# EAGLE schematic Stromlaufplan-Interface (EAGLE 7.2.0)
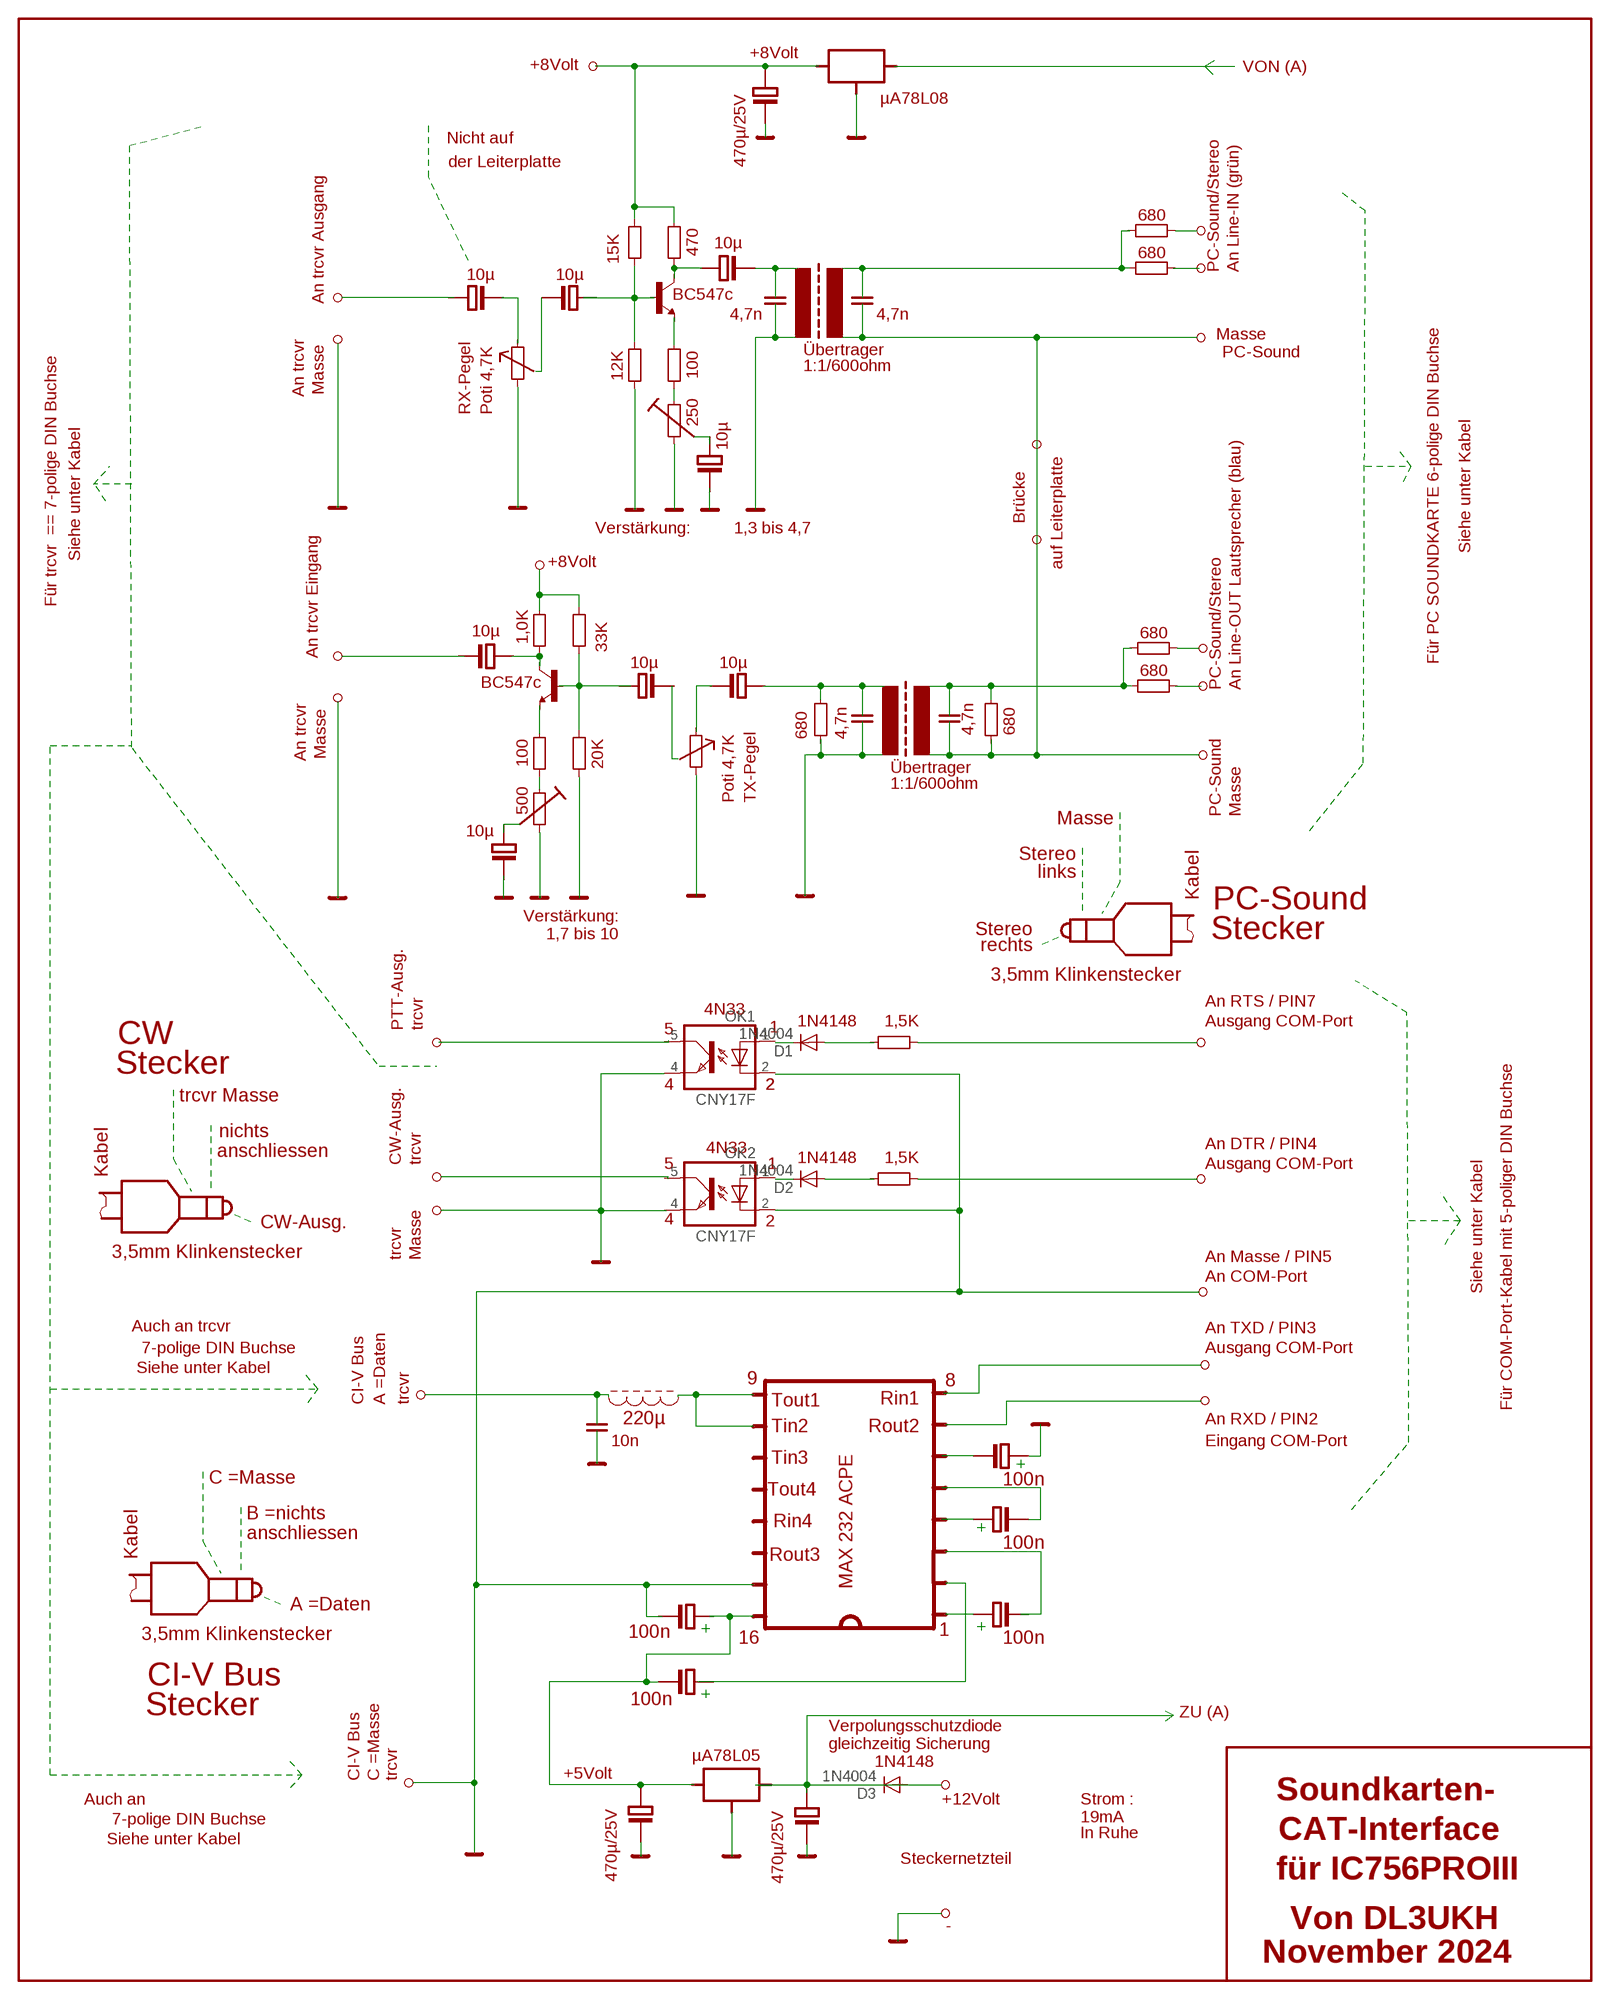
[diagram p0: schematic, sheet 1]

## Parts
D1  1N4004  [DO41-10]
D2  1N4004  [DO41-10]
D3  1N4004  [DO41-10]
OK1  CNY17F  [DIL06]
OK2  CNY17F  [DIL06]

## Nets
N$35: D3.C
N$45: D1.C
N$46: D1.A
N$47: D3.A
N$51: D2.C
N$55: D2.A
Unconnected: OK1.1(A) OK1.2(C) OK1.4(EMIT) OK1.5(COL) OK2.1(A) OK2.2(C) OK2.4(EMIT) OK2.5(COL)

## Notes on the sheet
- +8Volt
- +8Volt | VON (A)
- µA78L08
- Nicht auf
- der Leiterplatte | 470µ/25V
- 680
- 10µ
- 470 | 680
- 15K
- PC-Sound/Stereo | An Line-IN (grün)
- 10µ | 10µ
- An trcvr Ausgang | BC547c
- 4,7n | 4,7n
- Masse
- PC-Sound
- Übertrager
- 1:1/600ohm
- 12K | 100
- An trcvr | Masse
- RX-Pegel | Poti 4,7K
- 250
- 10µ
- Brücke
- Verstärkung: | 1,3 bis 4,7
- Siehe unter Kabel
- Siehe unter Kabel
- +8Volt | auf Leiterplatte
- Für trcvr  == 7-polige DIN Buchse
- 10µ | 680
- 1,0K
- 33K
- An trcvr Eingang
- 10µ | 10µ | Für PC SOUNDKARTE 6-polige DIN Buchse
- 680
- BC547c | PC-Sound/Stereo | An Line-OUT Lautsprecher (blau)
- 680 | 4,7n | 4,7n | 680
- An trcvr | Masse
- 100 | 20K
- Übertrager
- 1:1/600ohm
- Poti 4,7K | TX-Pegel
- 500 | PC-Sound | Masse
- Masse
- 10µ
- Stereo
- links
- Kabel
- PC-Sound
- Verstärkung:
- 1,7 bis 10 | Stereo | Stecker
- rechts
- 3,5mm Klinkenstecker
- An RTS / PIN7
- 4N33
- PTT-Ausg. | trcvr | 1N4148 | 1,5K | Ausgang COM-Port
- 5 | 1
- CW
- Stecker
- 4 | 2 | 2
- trcvr Masse
- nichts
- 4N33 | An DTR / PIN4
- anschliessen
- CW-Ausg. | trcvr | 1N4148 | 1,5K
- 5 | 1 | Ausgang COM-Port
- Kabel
- CW-Ausg. | 4 | 2
- 3,5mm Klinkenstecker | trcvr | Masse | An Masse / PIN5
- An COM-Port
- Siehe unter Kabel
- Auch an trcvr
- An TXD / PIN3
- 7-polige DIN Buchse
- Ausgang COM-Port
- Siehe unter Kabel
- 9 | 8
- CI-V Bus | A =Daten | trcvr | Tout1 | Rin1
- Für COM-Port-Kabel mit 5-poliger DIN Buchse
- 220µ | An RXD / PIN2
- Tin2 | Rout2
- 10n | Eingang COM-Port
- Tin3
- 100n
- C =Masse
- Tout4
- B =nichts
- Rin4
- anschliessen | 100n
- Kabel | Rout3
- MAX 232 ACPE
- A =Daten
- 100n | 1
- 16 | 100n
- 3,5mm Klinkenstecker
- CI-V Bus
- 100n
- Stecker | ZU (A)
- Verpolungsschutzdiode
- gleichzeitig Sicherung
- µA78L05
- 1N4148
- CI-V Bus | C =Masse | trcvr | +5Volt
- Auch an
- +12Volt | Strom : | Soundkarten-
- 7-polige DIN Buchse
- 19mA
- Siehe unter Kabel
- In Ruhe | CAT-Interface
- Steckernetzteil
- 470µ/25V | 470µ/25V | für IC756PROIII
- - | Von DL3UKH
- November 2024

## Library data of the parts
D1-D3 = diode:1N4004: DIODE
OK1 OK2 = optocoupler:CNY17F: SIEMENS OPTO COUPLER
